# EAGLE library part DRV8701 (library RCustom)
This is the DRV8701, one of TI's gate drivers to make a full bridge for motor control. Includes current sense logic inside with an external sense resistor.
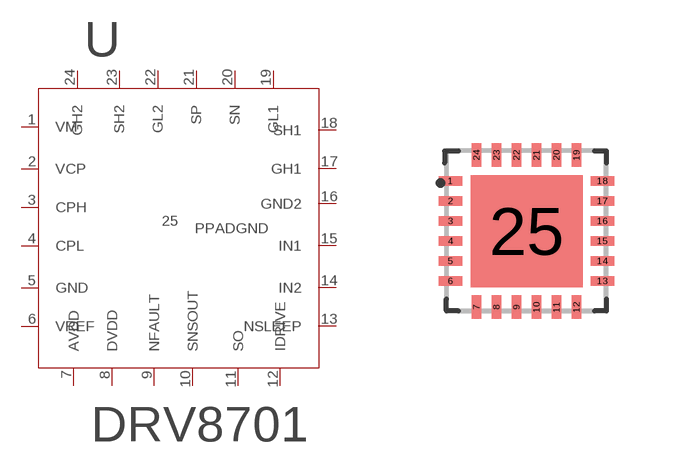
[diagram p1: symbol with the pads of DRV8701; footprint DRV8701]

Designator prefix U

## DRV8701  [DRV8701]
1  VM
2  VCP
3  CPH
4  CPL
5  GND
6  VREF
7  AVDD
8  DVDD
9  NFAULT
10  SNSOUT
11  SO
12  IDRIVE
13  NSLEEP
14  IN2
15  IN1
16  GND2
17  GH1
18  SH1
19  GL1
20  SN
21  SP
22  GL2
23  SH2
24  GH2
25  PPADGND

## Footprint DRV8701 (pad centres in mm)
smd 0.6 x 0.24: 1 -1.9,1.25; 2 -1.9,0.75; 3 -1.9,0.25; 4 -1.9,-0.25; 5 -1.9,-0.75; 6 -1.9,-1.25; 13 1.9,-1.25; 14 1.9,-0.75; 15 1.9,-0.25; 16 1.9,0.25; 17 1.9,0.75; 18 1.9,1.25
smd 0.24 x 0.6: 7 -1.25,-1.9; 8 -0.75,-1.9; 9 -0.25,-1.9; 10 0.25,-1.9; 11 0.75,-1.9; 12 1.25,-1.9; 19 1.25,1.9; 20 0.75,1.9; 21 0.25,1.9; 22 -0.25,1.9; 23 -0.75,1.9; 24 -1.25,1.9
smd 2.8 x 2.8: 25 0,0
